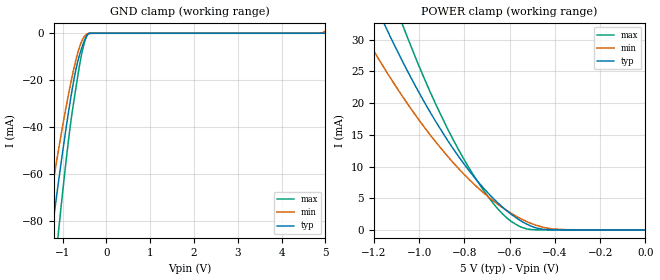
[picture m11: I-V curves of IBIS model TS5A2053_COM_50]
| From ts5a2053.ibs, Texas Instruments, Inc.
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[Model]   TS5A2053_COM_50
Model_type  Terminator
| variable   typ   min   max
C_comp   11.62pF   10.16pF   16.22pF
| C_tri-state   11.62pF   10.16pF   16.22pF
[Temperature Range]   40   100   -40
| Ambient temperature   25   85   -40
[Voltage range]   5   4.5   5.5
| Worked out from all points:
|   GND clamp passes 1 mA (typ) near -0.45 V on its own axis
|   POWER clamp passes 1 mA (typ) near -0.53 V on its own axis
[GND Clamp]
| TS5A2053_COM_50
|   Voltage   I(typ)   I(min)   I(max)
-5.5V     -821.7mA   -663.9mA   -1.071A
-1.42V    -110.6mA   -87.69mA   -146.3mA
-1.365V   -102.3mA   -81.03mA   -135.6mA
-1.255V   -86.11mA   -67.99mA   -114.4mA
-1.2V     -78.18mA   -61.63mA   -104mA
-1.105V   -64.81mA   -50.91mA   -86.48mA
-1.06V    -58.65mA   -45.98mA   -78.38mA
-830mV    -29.4mA    -22.68mA   -40.24mA
-655mV    -12.15mA   -8.428mA   -18.39mA
-525mV    -4.204mA   -2.015mA   -5.558mA
-400mV    -101.7uA   -68.88uA   -83.55uA
5V        690.3pA    962.1uA    4.599nA
[POWER Clamp]
| TS5A2053_COM_50
|   Voltage   I(typ)   I(min)   I(max)
-5.5V     713.2mA    553.4mA    953.5mA
-1.27V    41.77mA    32.53mA    52.71mA
-1.24V    39.28mA    30.65mA    49.36mA
-1.14V    31.43mA    24.72mA    38.84mA
-1.075V   26.7mA     21.15mA    32.53mA
-1.045V   24.62mA    19.58mA    29.77mA
-825mV    11.55mA    9.659mA    12.61mA
-720mV    6.79mA     6.003mA    6.491mA
-610mV    2.952mA    3.004mA    1.822mA
-545mV    1.317mA    1.672mA    394.9uA
-450mV    79.12uA    400.8uA    18.8uA
-95.1fV   690.3pA    4.86nA     16.88nA
